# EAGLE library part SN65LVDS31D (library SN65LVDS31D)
SN65LVDS31D, LVDS Transmitter Quad LVTTL 400Mbit/s, 3 3.6 V, 16-Pin, SOIC Source: Datasheet
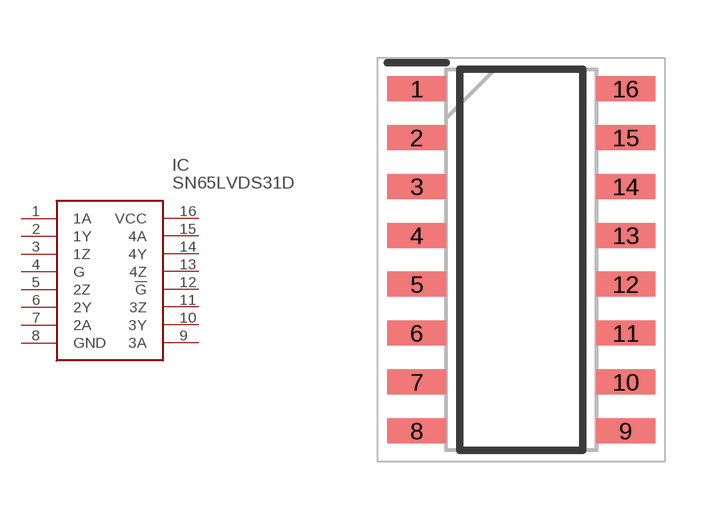
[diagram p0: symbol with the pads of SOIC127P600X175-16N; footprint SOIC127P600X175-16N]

Designator prefix IC

## SN65LVDS31D (Arrow_Part_Number: SN65LVDS31D; Arrow_Price-Stock: https://www.arrow.com/en/products/sn65lvds31d/texas-instruments?region=nac; Description: SN65LVDS31D, LVDS Transmitter Quad LVTTL 400Mbit/s, 3 3.6 V, 16-Pin, SOIC; Height: 1.75mm; Manufacturer_Name: Texas Instruments; Manufacturer_Part_Number: SN65LVDS31D; Mouser_Part_Number: 595-SN65LVDS31D; Mouser_Price-Stock: https://www.mouser.co.uk/ProductDetail/Texas-Instruments/SN65LVDS31D?qs=b0gIXGU74fMgoTCqNA4zrw%3D%3D)  [SOIC127P600X175-16N]
1  1A
2  1Y
3  1Z
4  G
5  2Z
6  2Y
7  2A
8  GND
9  3A
10  3Y
11  3Z
12  !G
13  4Z
14  4Y
15  4A
16  VCC

## Footprint SOIC127P600X175-16N (pad centres in mm)
D (R-PDSO-G16)
smd 1.525 x 0.65: 1 -2.712,4.445; 2 -2.712,3.175; 3 -2.712,1.905; 4 -2.712,0.635; 5 -2.712,-0.635; 6 -2.712,-1.905; 7 -2.712,-3.175; 8 -2.712,-4.445; 9 2.712,-4.445; 10 2.712,-3.175; 11 2.712,-1.905; 12 2.712,-0.635; 13 2.712,0.635; 14 2.712,1.905; 15 2.712,3.175; 16 2.712,4.445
